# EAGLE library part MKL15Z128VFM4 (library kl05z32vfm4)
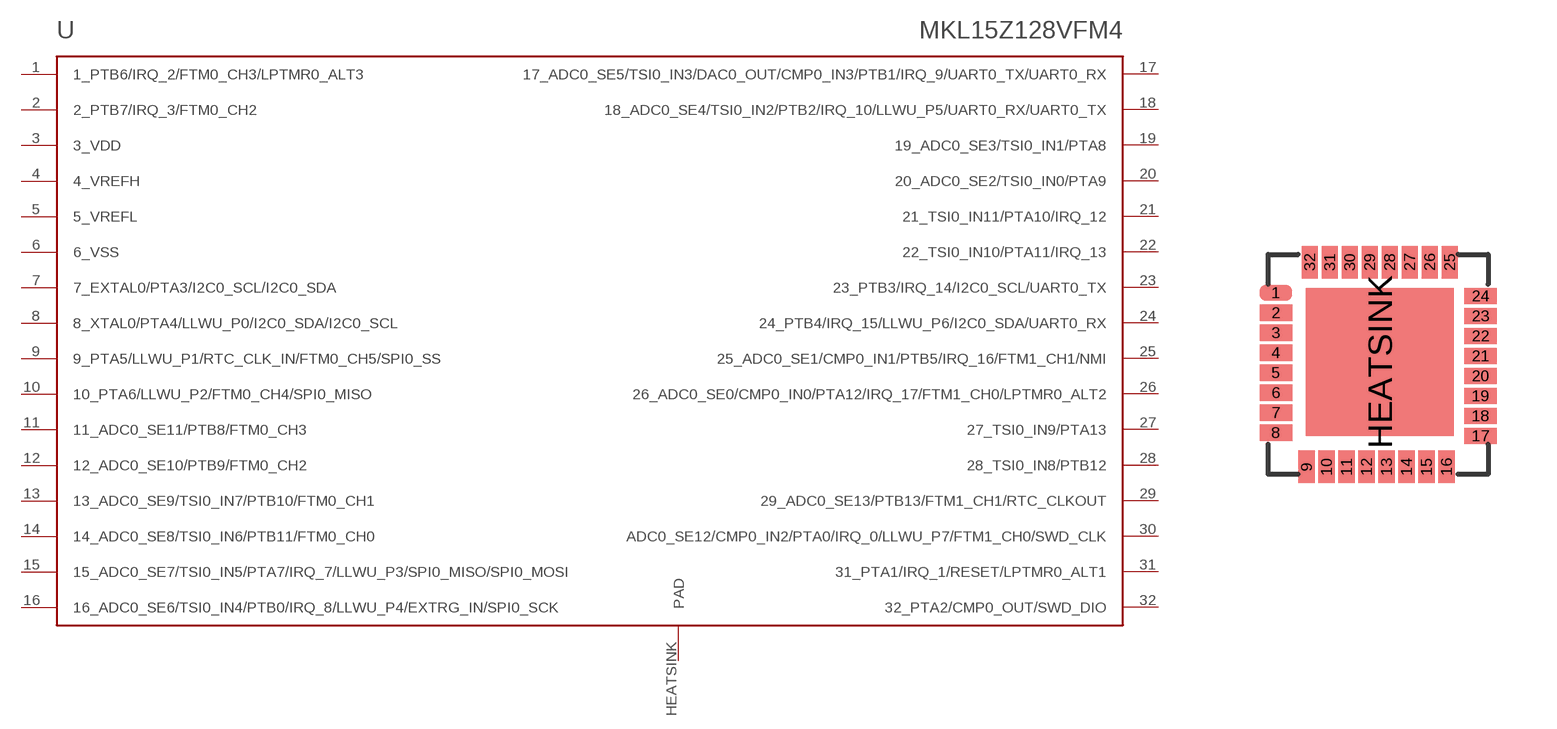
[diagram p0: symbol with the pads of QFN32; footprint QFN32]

Designator prefix -

## MKL15Z128VFM4  [QFN32]
1  1_PTB6/IRQ_2/FTM0_CH3/LPTMR0_ALT3
2  2_PTB7/IRQ_3/FTM0_CH2
3  3_VDD
4  4_VREFH
5  5_VREFL
6  6_VSS
7  7_EXTAL0/PTA3/I2C0_SCL/I2C0_SDA
8  8_XTAL0/PTA4/LLWU_P0/I2C0_SDA/I2C0_SCL
9  9_PTA5/LLWU_P1/RTC_CLK_IN/FTM0_CH5/SPI0_SS
10  10_PTA6/LLWU_P2/FTM0_CH4/SPI0_MISO
11  11_ADC0_SE11/PTB8/FTM0_CH3
12  12_ADC0_SE10/PTB9/FTM0_CH2
13  13_ADC0_SE9/TSI0_IN7/PTB10/FTM0_CH1
14  14_ADC0_SE8/TSI0_IN6/PTB11/FTM0_CH0
15  15_ADC0_SE7/TSI0_IN5/PTA7/IRQ_7/LLWU_P3/SPI0_MISO/SPI0_MOSI
16  16_ADC0_SE6/TSI0_IN4/PTB0/IRQ_8/LLWU_P4/EXTRG_IN/SPI0_SCK
17  17_ADC0_SE5/TSI0_IN3/DAC0_OUT/CMP0_IN3/PTB1/IRQ_9/UART0_TX/UART0_RX
18  18_ADC0_SE4/TSI0_IN2/PTB2/IRQ_10/LLWU_P5/UART0_RX/UART0_TX
19  19_ADC0_SE3/TSI0_IN1/PTA8
20  20_ADC0_SE2/TSI0_IN0/PTA9
21  21_TSI0_IN11/PTA10/IRQ_12
22  22_TSI0_IN10/PTA11/IRQ_13
23  23_PTB3/IRQ_14/I2C0_SCL/UART0_TX
24  24_PTB4/IRQ_15/LLWU_P6/I2C0_SDA/UART0_RX
25  25_ADC0_SE1/CMP0_IN1/PTB5/IRQ_16/FTM1_CH1/NMI
26  26_ADC0_SE0/CMP0_IN0/PTA12/IRQ_17/FTM1_CH0/LPTMR0_ALT2
27  27_TSI0_IN9/PTA13
28  28_TSI0_IN8/PTB12
29  29_ADC0_SE13/PTB13/FTM1_CH1/RTC_CLKOUT
30  ADC0_SE12/CMP0_IN2/PTA0/IRQ_0/LLWU_P7/FTM1_CH0/SWD_CLK
31  31_PTA1/IRQ_1/RESET/LPTMR0_ALT1
32  32_PTA2/CMP0_OUT/SWD_DIO
HEATSINK  PAD

## Footprint QFN32 (pad centres in mm)
smd 0.813 x 0.406: 1 -2.56,1.79; 2 -2.56,1.29; 3 -2.56,0.79; 4 -2.56,0.29; 5 -2.56,-0.21; 6 -2.56,-0.71; 7 -2.56,-1.21; 8 -2.56,-1.71; 17 2.56,-1.79; 18 2.56,-1.29; 19 2.56,-0.79; 20 2.56,-0.29; 21 2.56,0.21; 22 2.56,0.71; 23 2.56,1.21; 24 2.56,1.71
smd 0.406 x 0.813: 9 -1.79,-2.56; 10 -1.29,-2.56; 11 -0.79,-2.56; 12 -0.29,-2.56; 13 0.21,-2.56; 14 0.71,-2.56; 15 1.21,-2.56; 16 1.71,-2.56; 25 1.79,2.56; 26 1.29,2.56; 27 0.79,2.56; 28 0.29,2.56; 29 -0.21,2.56; 30 -0.71,2.56; 31 -1.21,2.56; 32 -1.71,2.56
smd 3.7 x 3.7: HEATSINK 0.04,0.06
